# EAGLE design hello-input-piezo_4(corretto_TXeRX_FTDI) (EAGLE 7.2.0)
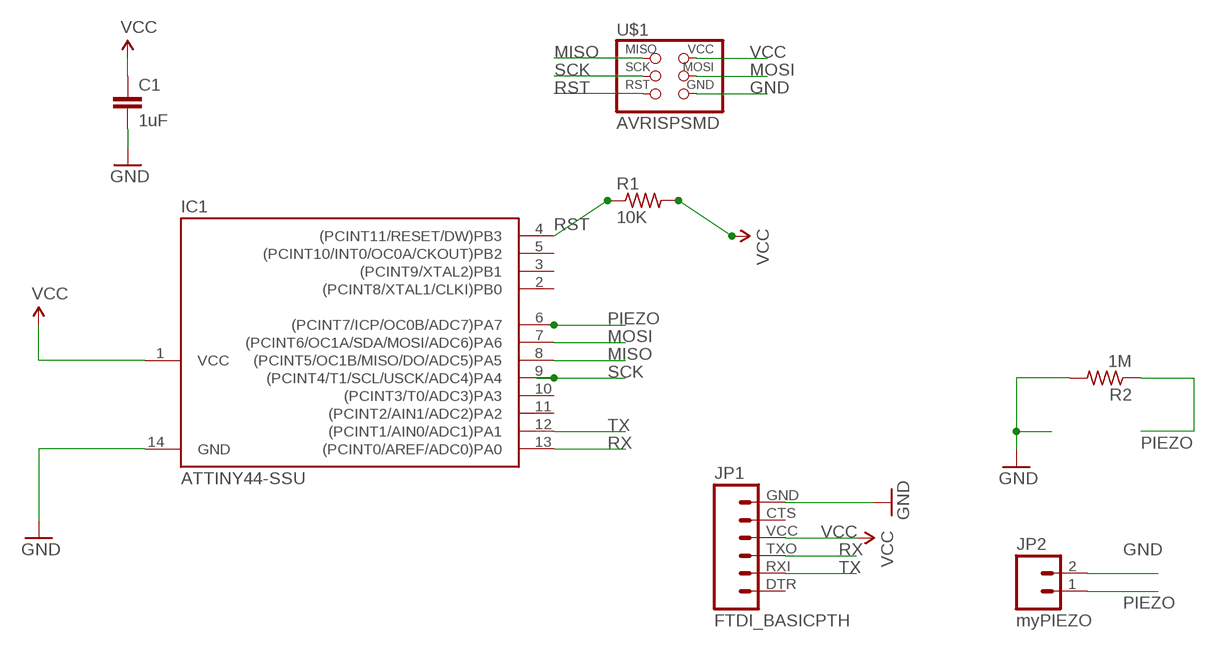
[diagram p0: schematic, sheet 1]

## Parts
C1  1uF  CAP1206  [1206]
IC1  ATTINY44-SSU  [SOIC14]
JP1  FTDI_BASICPTH  [FTDI_BASIC]
JP2  myPIEZO  M02LOCK_LONGPADS  [1X02_LOCK_LONGPADS]
R1  10K  RES-US1206  [R1206]
R2  1M  RES-US1206  [R1206]
U$1  AVRISPSMD  [2X03SMD]

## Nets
GND: C1.2 IC1.14(GND) JP1.GND JP2.2 R2.2 U$1.6(GND)
MISO: IC1.8((PCINT5/OC1B/MISO/DO/ADC5)PA5) U$1.1(MISO)
MOSI: IC1.7((PCINT6/OC1A/SDA/MOSI/ADC6)PA6) U$1.4(MOSI)
PIEZO: IC1.6((PCINT7/ICP/OC0B/ADC7)PA7) JP2.1 R2.1
RST: IC1.4((PCINT11/RESET/DW)PB3) R1.1 U$1.5(RST)
RX: IC1.13((PCINT0/AREF/ADC0)PA0) JP1.TXO
SCK: IC1.9((PCINT4/T1/SCL/USCK/ADC4)PA4) U$1.3(SCK)
TX: IC1.12((PCINT1/AIN0/ADC1)PA1) JP1.RXI
VCC: C1.1 IC1.1(VCC) JP1.VCC R1.2 U$1.2(VCC)
Unconnected: IC1.2((PCINT8/XTAL1/CLKI)PB0) IC1.3((PCINT9/XTAL2)PB1) IC1.5((PCINT10/INT0/OC0A/CKOUT)PB2) IC1.10((PCINT3/T0/ADC3)PA3) IC1.11((PCINT2/AIN1/ADC2)PA2) JP1.CTS JP1.DTR

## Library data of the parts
C1 = SparkFun-Passives:CAP: Capacitor
IC1 = fab:ATTINY44
JP1 = SparkFun-Connectors:FTDI_BASIC: FTDI Basic header with labels
JP2 = SparkFun-Connectors:M02: Standard 2-pin 0.1" header. Use with
R1 R2 = fab:RES-US: Resistor (US Symbol)
U$1 = fab:AVRISP

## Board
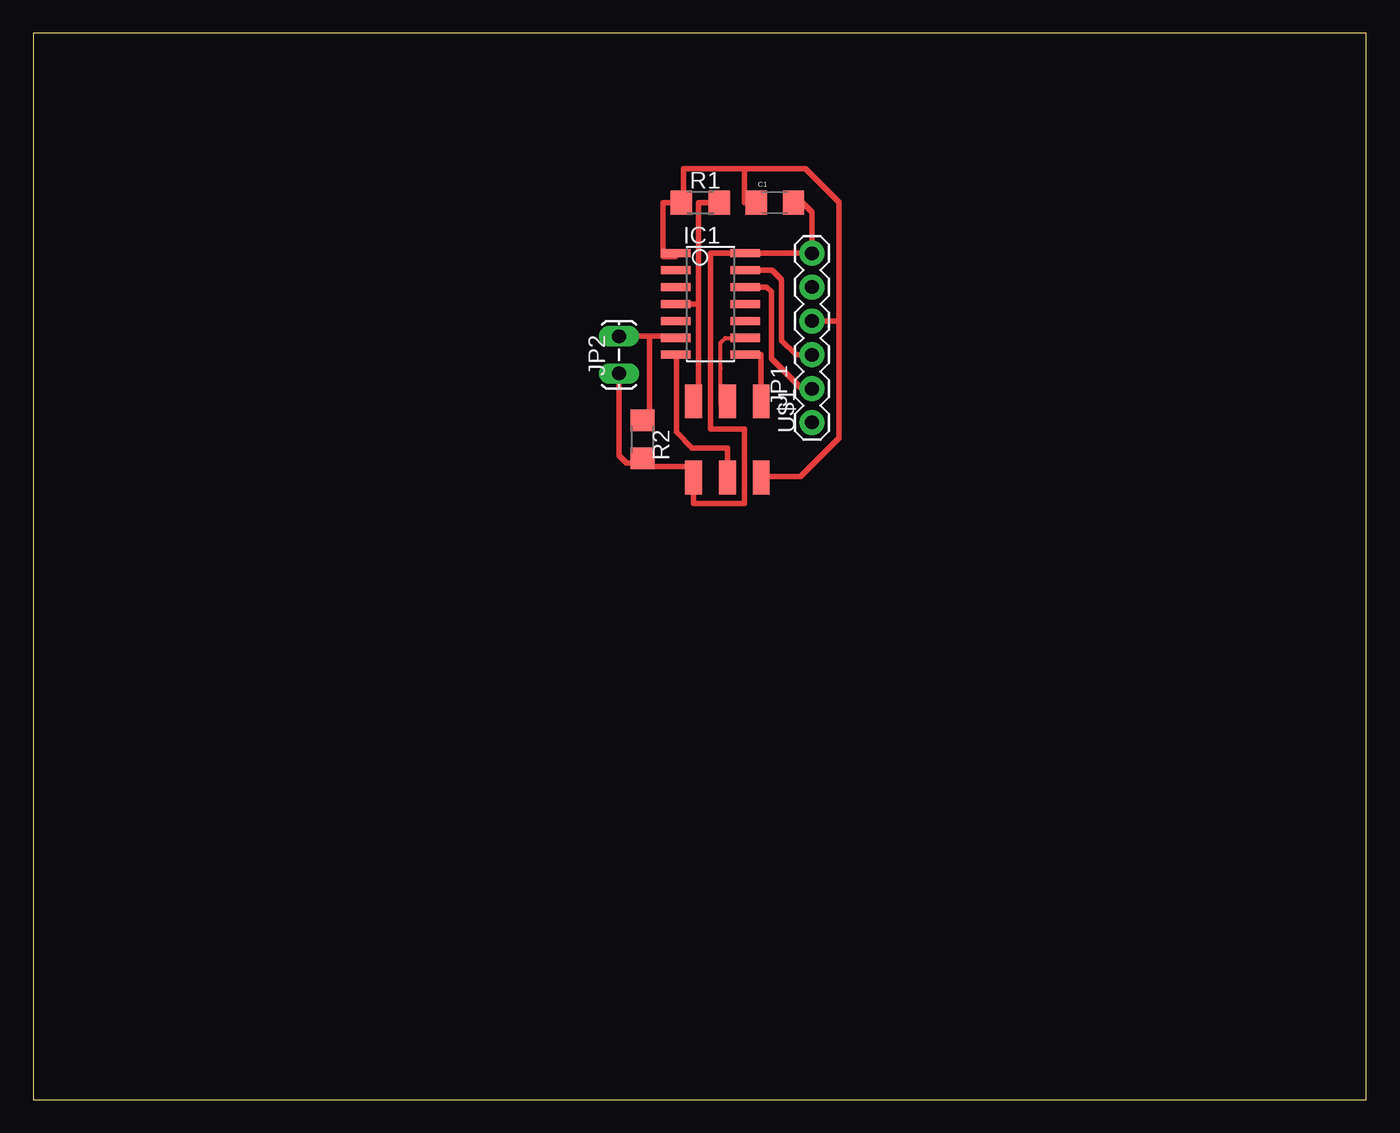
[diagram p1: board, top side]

Size 100 x 80 mm. Coordinates in mm from the lower left corner, seen from the top.
Outline: 0,0 100,0 100,80 0,80 0,0
Copper layers (1*16): Top 0.035mm / dielectric 1.5mm / Bottom 0.035mm
Design rules "default": minimum track width 10mil, minimum drill 24mil, track to track 8mil, track to pad 8mil, pad to pad 8mil, via to via 8mil, smd to smd 8mil, copper to edge 40mil, drill to drill 8mil, minimum pad ring 10mil, minimum via ring 8mil, stop-mask expansion 4mil, vias tented up to drill 0mil, thermal gap 10mil

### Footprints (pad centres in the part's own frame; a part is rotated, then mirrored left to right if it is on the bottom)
1206 = smd 1.6 x 1.8: 1 -1.4,0; 2 1.4,0
SOIC14 = smd 0.61 x 2.21: 1 -3.81,-2.603; 2 -2.54,-2.603; 3 -1.27,-2.603; 4 0,-2.603; 5 1.27,-2.603; 6 2.54,-2.603; 7 3.81,-2.603; 8 3.81,2.603; 9 2.54,2.603; 10 1.27,2.603; 11 0,2.603; 12 -1.27,2.603; 13 -2.54,2.603; 14 -3.81,2.603
FTDI_BASIC = drill 1.016 pad 1.88: CTS 10.16,0; DTR 0,0; GND 12.7,0; RXI 2.54,0; TXO 5.08,0; VCC 7.62,0
1X02_LOCK_LONGPADS = drill 1.016 long: 1 -0.127,0; 2 2.667,0
R1206 = smd 1.6 x 1.803: 1 -1.422,0; 2 1.422,0
2X03SMD = smd 2.54 x 1.27: 1 -2.857,2.54; 2 2.857,2.54; 3 -2.857,0; 4 2.857,0; 5 -2.857,-2.54; 6 2.857,-2.54

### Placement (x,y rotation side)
C1  55.63,67.31 0 top
IC1  50.8,59.69 270 top
JP1  58.42,50.8 90 top
JP2  43.94,57.15 270 top
R1  50.04,67.31 180 top
R2  45.72,49.53 270 top
U$1  52.07,49.53 270 top

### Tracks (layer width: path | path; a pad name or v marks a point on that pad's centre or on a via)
GND
  Top 0.406: U$1.6 49.53,44.7 53.34,44.7 53.34,50.29 50.8,50.29 50.8,63.5 IC1.14 JP1.GND 58.42,66.59 57.7,67.31 C1.2 | U$1.6 49.53,47.5 45.21,47.5 45.21,47.75 | 49.53,46.48 U$1.6 | JP2.2 43.94,48.32 44.51,47.75 45.21,47.75 | 45.21,47.75 45.72,47.75 R2.2
MISO
  Top 0.406: U$1.1 54.61,55.88 IC1.8 53.34,55.88
MOSI
  Top 0.406: IC1.7 48.26,55.88 48.26,50.07 49.43,48.9 52.07,48.9 U$1.4
PIEZO
  Top 0.406: 48.2,57.05 IC1.6 48.2,57.28 46.23,57.28 | 46.23,57.28 JP2.1 | R2.1 46.23,50.95 46.23,57.28
RST
  Top 0.406: R1.1 49.91,67.31 49.91,59.69 | IC1.4 49.91,59.69 | 49.91,59.69 49.91,52.7 49.53,52.7 U$1.5
RX
  Top 0.406: IC1.13 55.42,62.23 56.13,61.51 56.13,56.96 57.21,55.88 JP1.TXO
SCK
  Top 0.305: U$1.3 51.56,52.07 51.56,53.59 51.56,54.86 51.56,56.79 51.92,57.15 IC1.9
TX
  Top 0.406: IC1.12 55.01,60.96 55.37,60.6 55.37,55.58 56.09,54.86 56.64,54.31 57.61,53.34 JP1.RXI
VCC
  Top 0.406: C1.1 53.34,67.31 53.34,69.85 | 60.45,58.42 60.45,49.63 57.56,46.74 54.61,46.74 U$1.2 | 53.34,69.85 57.94,69.85 60.45,67.34 60.45,58.42 | JP1.VCC 60.45,58.42 | 53.34,69.85 48.77,69.85 48.77,67.31 R1.2 47.24,67.31 47.24,63.25 48.2,63.25 IC1.1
